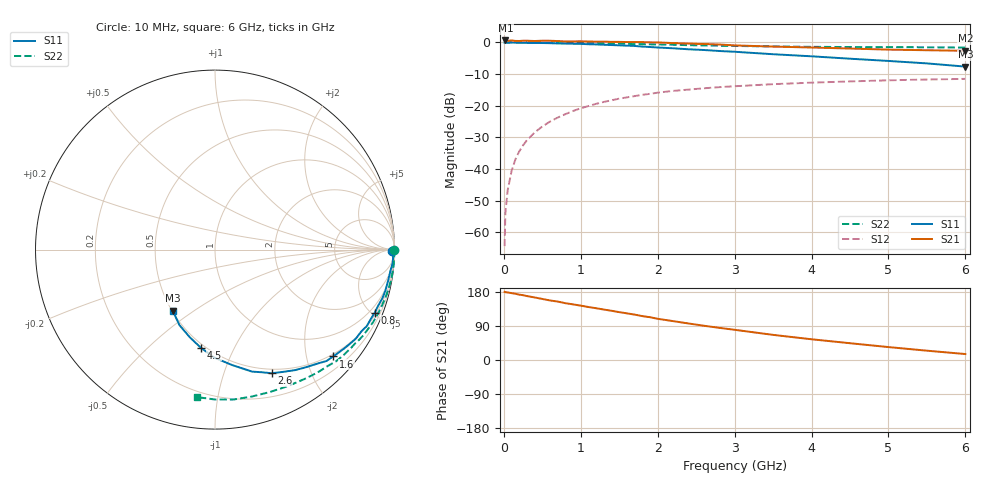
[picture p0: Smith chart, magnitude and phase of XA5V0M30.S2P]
! SIEMENS Discrete & RF Semiconductors
! BFY180
! Si NPN RF Bipolar Junction Transistor in MICRO-X
! VCE = 5 V  IC = 0.3 mA
! Common Emitter S-Parameters:  May  1997
# GHz  S  MA  R  50
!  f  S11  S21  S12  S22
! GHz  MAG  ANG  MAG  ANG  MAG  ANG  MAG  ANG
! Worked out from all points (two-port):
!   36 points, 10 MHz to 6 GHz, reference 50 ohm
!   highest |S21| = 0.60 dB at 20 MHz (marker M1); lowest = -2.7 dB at 6 GHz (marker M2)
!   |S21| within 3 dB of the highest: start of sweep to 5.266 GHz
!   lowest |S11| = -7.7 dB at 6 GHz (marker M3), VSWR 2.41, Z = 25.2 - j20.7 ohm
!   |S11| at or under -10 dB: nowhere
!   |S22| runs from -1.6 to 0.0 dB; largest |S21 - S12| = 1.1
!   S11 on the Smith chart (normalised r, x): 10 MHz: open; 800 MHz: 0.62, -5.20; 1.6 GHz: 0.45, -2.53; 2.6 GHz: 0.45, -1.46; 4.5 GHz: 0.48, -0.75; 6 GHz: 0.50, -0.41
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0.01  0.9874 -0.4  1.055 179.7  0.0006 94.4  0.9992 -0.2
0.02  0.9866 -0.6  1.072 179.0  0.002 88.1  0.9999 -0.4
0.05  0.9883 -1.3  1.054 178.2  0.0046 89.6  0.999 -1.0
0.1  0.9934 -2.6  1.072 176.5  0.0092 88.7  0.9991 -2.1
0.15  0.9923 -4.4  1.054 174.8  0.0141 86.4  0.9999 -3.2
0.2  0.989 -5.4  1.052 172.5  0.0189 85.5  0.9986 -4.1
0.3  0.9829 -8.0  1.062 168.7  0.0284 83.5  0.9974 -6.2
0.4  0.9792 -10.7  1.051 165.1  0.0376 81.5  0.9969 -8.2
0.6  0.9713 -16.2  1.061 157.1  0.0559 76.7  0.9911 -12.4
0.8  0.957 -21.5  1.034 149.9  0.0733 72.1  0.985 -16.5
1.1  0.934 -29.2  1.032 139.8  0.0985 65.3  0.9733 -22.5
1.3  0.9172 -34.8  1.028 133.1  0.1145 60.9  0.9635 -26.5
1.6  0.8877 -42.1  1.012 123.1  0.1351 54.9  0.9468 -32.2
2  0.8295 -52.1  0.998 108.7  0.1603 47.2  0.927 -39.3
2.2  0.8063 -56.4  0.974 102.6  0.171 43.4  0.9173 -42.8
2.6  0.7576 -65.4  0.942 90.4  0.188 37.0  0.894 -49.2
2.8  0.7303 -69.3  0.925 84.9  0.1959 33.9  0.8851 -52.2
3.5  0.6494 -81.7  0.858 66.3  0.2184 24.5  0.8619 -62.1
4  0.6021 -90.3  0.829 54.7  0.2308 18.3  0.8503 -69.0
4.5  0.5517 -98.3  0.799 44.3  0.2413 12.7  0.844 -75.9
5.5  0.4651 -115.2  0.751 24.6  0.2588 2.1  0.8352 -90.0
6  0.4137 -124.8  0.735 15.7  0.2649 -3.4  0.8278 -97.1
